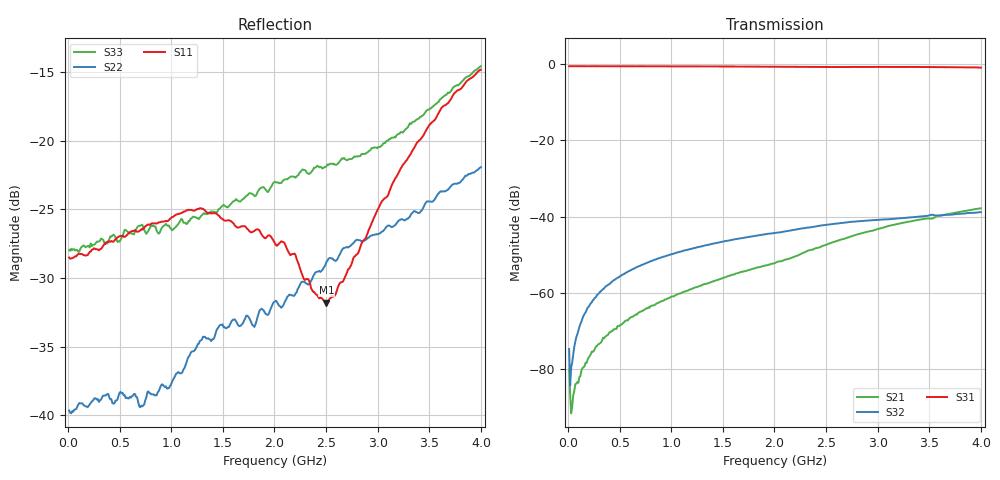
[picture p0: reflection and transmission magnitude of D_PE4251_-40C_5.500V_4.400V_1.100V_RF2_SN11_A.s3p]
! Device ID: PE4251_SoldCshunt_081809
! Dir: c:\Test Bench Repositories\Bench_Software_CVI_Version_8\trunk\PSC 4Port_VNA Bench\datalog\4250\TEST\PE4251_SoldCshunt_081809\-40C\5p500000\RF2
! Serial: 11
! Insertion: A
! Temp: -40C
! VDD: 5.500
! Control_Hi: 80.000
! Control_Lo: 20.000
! Logic State: RF2
! Port 1: RFC
! Port 2: RF1
! Port 3: RF2
! V1 = 1.10
! V2 = 1.10
! V3 = 1.10
! IDD: 6.462750e-05
! FILE NAME
! DATE 08/18/09  20:11
! CORRECTED  DATA
#  Hz  S  RI  R  50.00
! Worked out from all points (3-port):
!   401 points, 10 MHz to 4 GHz, reference 50 ohm
!   strongest paths, dB at 10 MHz, 1.008 GHz, 2.005 GHz, 3.002 GHz, 4 GHz:
!     S31: -0.5, -0.5, -0.6, -0.7, -0.8
!     S32: -74.8, -49.9, -44.3, -40.9, -38.8
!     S21: -80.2, -61.0, -52.2, -43.3, -37.8
!   lowest |S11| = -31.8 dB at 2.504 GHz (marker M1), VSWR 1.05, Z = 50.6 - j2.53 ohm
!   |S11| at or under -10 dB: start of sweep to end of sweep
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1e7  0.0375 -0.000729  -2.91e-05 -4e-05  0.945 -0.00273
     1.1e-05 -9.67e-05  0.0104 -0.000724  1.33e-05 -9.03e-07
     0.9456 -0.00431  0.000179 3.39e-05  0.04 0.000331
3.9925e7  0.0373 0.000616  2.3e-05 -3.9e-05  0.9461 -0.0159
          1.83e-05 -2.61e-05  0.0103 -0.000208  2.36e-05 0.000119
          0.9467 -0.0156  1.58e-05 0.00012  0.0399 0.000113
8.98e7  0.0384 0.0017  1.39e-05 -6.35e-05  0.9458 -0.0323
        1.2e-05 -6.63e-05  0.0108 5.73e-06  2.71e-05 0.000291
        0.9465 -0.0326  3.06e-05 0.000283  0.0399 -0.000705
1.696e8  0.038 0.00324  -1.22e-05 -0.000117  0.9429 -0.0596
         -8.16e-06 -0.00012  0.0107 0.00135  3.89e-05 0.000562
         0.9437 -0.06  3.29e-05 0.000551  0.0409 0.00164
5.0875e8  0.0447 0.00532  -0.000198 -0.00033  0.9263 -0.1755
          -0.000192 -0.000328  0.0116 0.00364  0.000152 0.00165
          0.9269 -0.1748  0.000157 0.00165  0.0435 -0.00202
7.18225e8  0.0473 0.0025  -0.000388 -0.000417  0.9101 -0.2446
           -0.000393 -0.000422  0.0101 0.00372  0.000283 0.00231
           0.9113 -0.2446  0.000282 0.00231  0.0492 -0.00519
1.2868e9  0.0561 -0.00868  -0.00112 -0.000547  0.8368 -0.4227
          -0.00111 -0.000537  0.0169 0.00804  0.000708 0.00399
          0.8399 -0.4228  0.000708 0.00398  0.0524 -0.00857
2.005e9  0.038 -0.0183  -0.00234 -0.000753  0.7009 -0.6083
         -0.00232 -0.000756  0.0166 0.02  0.00129 0.00596
         0.7037 -0.6082  0.00128 0.00597  0.0648 -0.0286
2.50375e9  0.00628 -0.025  -0.00411 -0.00124  0.591 -0.7082
           -0.00409 -0.00124  0.0185 0.0311  0.00178 0.00759
           0.5932 -0.7077  0.00179 0.0076  0.0531 -0.0609
4e9  -0.1799 -0.0219  -0.0127 0.00261  0.1351 -0.8983
     -0.0126 0.0026  -0.0292 0.0746  0.00292 0.011
     0.1363 -0.8968  0.0029 0.0111  -0.1284 -0.1354
